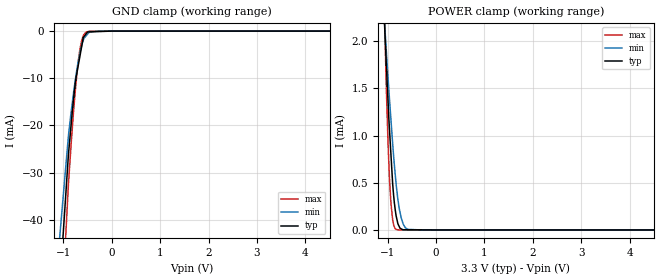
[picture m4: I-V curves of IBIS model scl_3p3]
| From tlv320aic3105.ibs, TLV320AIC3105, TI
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|   scl_3p3 Model
[Model]   scl_3p3
Model_type   Input
Vinl = 0.99
Vinh = 2.31
|   typ   min   max
|   (nom PVT)   (fast PVT)   (slow PVT)
C_comp   1.114e-12   1.105e-12   1.129e-12
| Where nom  PVT is Nominal Process, 3.3V, 27C
|   Fast PVT is Strong Process,  3.6V, -40C
|   Slow PVT is Weak Process,   2.7V, 105C
[Model Spec]
|Subparameter   typ   min   max
Vinh   2.31   1.89   2.52
Vinl   0.99   0.81   1.08
[Voltage Range]   3.3   2.7   3.6
|Ambient Temperature   25   85   -40
|Junction Temperature
[Temperature Range]   27   105   -40
[Power Clamp Reference]   3.3   2.7   3.6
[GND Clamp Reference]   0   0   0
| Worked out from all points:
|   GND clamp passes 1 mA (typ) near -0.56 V on its own axis
|   POWER clamp passes 1 mA (typ) near -0.96 V on its own axis
[GND Clamp]
|   Voltage   I(typ)   I(min)   I(max)
-3.3V     -1.745A    -1.522A    -1.934A
-1.494V   -118.7mA   -93.16mA   -148.6mA
-897.6mV  -26.09mA   -22.13mA   -32.42mA
-842.4mV  -19.83mA   -17.17mA   -23.94mA
-772.2mV  -12.51mA   -11.53mA   -14.59mA
-745.8mV  -10.15mA   -9.639mA   -11.43mA
-702mV    -7.665mA   -6.818mA   -7.047mA
-622.8mV  -3.177mA   -2.974mA   -1.957mA
-590.7mV  -1.359mA   -1.919mA   -1.016mA
-532.8mV  -597.9uA   -1.011mA   -208.3uA
-286.2mV  -107.2uA   -2.585uA   -6.129uA
6.6V      0A         0A         0A
[POWER Clamp]
|   Voltage   I(typ)   I(min)   I(max)
-3.3V     32.15mA    22.38mA    56.05mA
-1.076V   2.305mA    2.283mA    2.475mA
-1.03V    1.766mA    1.906mA    1.532mA
-993.6mV  1.375mA    1.621mA    934uA
-964.8mV  1.081mA    1.4mA      561.5uA
-932.4mV  796.9uA    1.166mA    280.4uA
-881.1mV  387.7uA    807.4uA    64.82uA
-820.8mV  138.7uA    461.6uA    4.877uA
-766.8mV  41.34uA    246.3uA    409.3nA
-718.2mV  11.1uA     124.3uA    128.1nA
-583.2mV  2.076uA    6.133uA    0A
6.6V      0A         0A         0A
